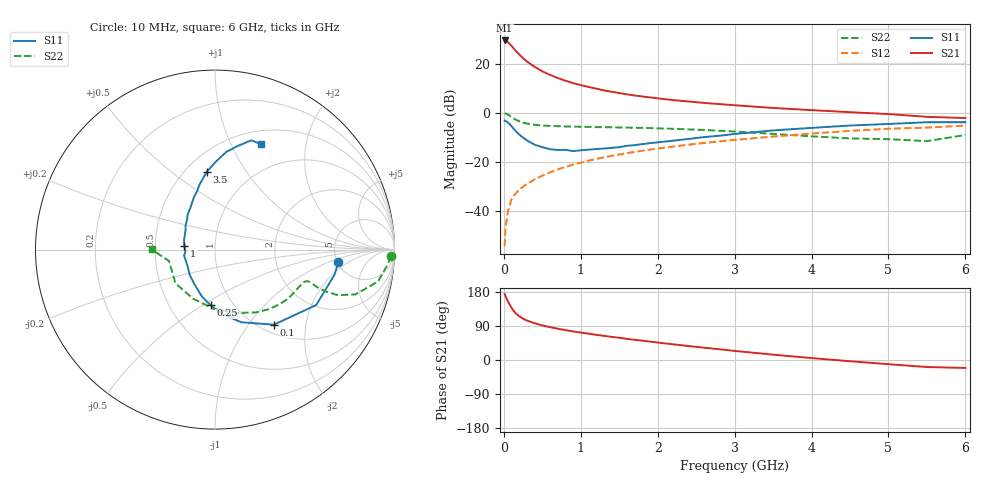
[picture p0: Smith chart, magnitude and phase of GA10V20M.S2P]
! Infineon Technologies  Discrete & RF Semiconductors
! BF775
! Si NPN RF Bipolar Junction Transistor in SOT23
! VCE = 10 V  IC = 20 mA
! Common Emitter S-Parameters:  May  1996
# GHz  S  MA  R  50
!  f  S11  S21  S12  S22
! GHz  MAG  ANG  MAG  ANG  MAG  ANG  MAG  ANG
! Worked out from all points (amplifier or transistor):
!   36 points, 10 MHz to 6 GHz, reference 50 ohm
!   highest |S21| = 29.5 dB at 10 MHz (marker M1)
!   |S21| within 3 dB of that: start of sweep to 121.4 MHz
!   unconditionally stable (mu >= 1): 458.3 MHz to 2.602 GHz
!   at 250 MHz: K = 0.81, MSG = 26.2 dB, |S12| = -30.2 dB
!   at 1.4 GHz: K = 1.09, MAG = 11.2 dB, |S12| = -17.6 dB
!   at 6 GHz: K = 0.88, MSG = 1.5 dB, |S12| = -5.2 dB
!   S11 on the Smith chart (normalised r, x): 10 MHz: 5.09, -1.38; 100 MHz: 1.15, -1.34; 250 MHz: 0.79, -0.54; 1 GHz: 0.71, +0.03; 3.5 GHz: 0.63, +0.68; 6 GHz: 0.66, +1.31
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0.01  0.6912 -5.9  29.86 174.3  0.0019 88.9  0.9796 -2.1
0.02  0.6803 -11.9  29.45 169.4  0.0041 78.4  0.968 -4.6
0.05  0.643 -28.7  27.86 155.8  0.0093 76.3  0.9256 -11.1
0.1  0.5315 -51.9  23.15 137.6  0.0172 69.1  0.8211 -17.7
0.15  0.4301 -70.2  18.72 124.0  0.0223 65.7  0.7312 -20.3
0.2  0.3611 -83.9  15.46 115.5  0.0271 65.9  0.6706 -20.7
0.25  0.3109 -94.6  12.95 109.0  0.031 65.9  0.6298 -20.5
0.3  0.2727 -105.3  11.14 104.1  0.0354 67.3  0.6028 -20.1
0.4  0.2231 -121.3  8.644 97.1  0.0435 68.3  0.5696 -19.1
0.5  0.1986 -135.4  7.006 91.2  0.0521 69.5  0.5498 -18.8
0.6  0.1804 -146.9  5.925 86.7  0.0608 69.9  0.5399 -19.0
0.7  0.174 -159.2  5.131 82.6  0.0697 70.6  0.5326 -19.5
0.8  0.1756 -168.6  4.505 78.8  0.0784 70.3  0.5265 -20.1
1  0.1716 173.5  3.665 72.4  0.096 69.9  0.5184 -21.9
1.1  0.1767 167.4  3.363 69.5  0.1053 69.4  0.5148 -23.3
1.3  0.1863 154.6  2.868 63.8  0.1234 68.0  0.5075 -25.7
1.6  0.212 140.7  2.377 55.7  0.1499 66.0  0.4971 -30.0
2.2  0.2692 120.8  1.814 41.4  0.2046 61.0  0.4716 -40.1
3.5  0.4366 96.0  1.255 14.1  0.3274 47.3  0.3713 -71.9
4.5  0.549 83.3  1.029 -3.3  0.427 34.9  0.2997 -113.9
5.5  0.641 71.7  0.826 -18.5  0.4984 19.3  0.2638 -165.9
6  0.6412 66.4  0.781 -21.0  0.5481 14.9  0.3524 179.9
